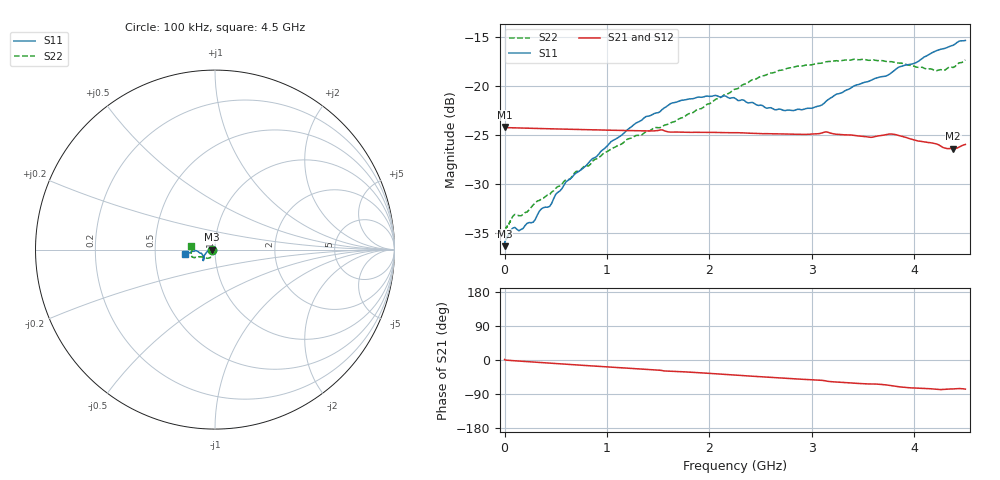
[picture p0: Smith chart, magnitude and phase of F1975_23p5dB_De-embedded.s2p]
! Integrated Device Technology
! Corporate Headquarters
! 6024 Silver Creek Valley Road
! San Jose, CA 95138  USA
! Phone:  1-408-284-8200
! Toll Free:  1-800-223-1366
! Webpage:  http://www.idt.com/
! Timing and RF Division
! 515 Groton Road, Suite 102
! Westford, MA 01886-6024
! Device:  F1975
! Description: 6-bit, 75 ohm, 0.5 dB Digital Step Attenuator
! Frequency:  5.0 MHz -  3.00 GHz
! Package:  4x4 mm QFN Plastic Package: 20 pin
! Ports:  2 RF, 11 DC
!  Pin  1  = D5 (16 dB)
!  Pin  2  = RF1  =  Port 1
!  Pin  3  = Serial Data In (DATA)
!  Pin  4  = Serial Clock (CLK)
!  Pin  5  = Serial Latch Enable (LE)
!  Pin  6  = VDD
!  Pin  7  = NC
!  Pin  8  = NC
!  Pin  9  = NC
!  Pin 10  = GND
!  Pin 11  = GND
!  Pin 12  = NC
!  Pin 13  = VMODE
!  Pin 14  = RF2  =  Port 2
!  Pin 15  = D4 (8 dB)
!  Pin 16  = D3 (4 dB)
!  Pin 17  = D2 (2 dB)
!  Pin 18  = NC
!  Pin 19  = D1 (1 dB)
!  Pin 20  = D0 (0.5 dB)
! State:  47
! Atten State:  23.5 dB
! Voltage:  +3.30 Volts
! Current:  0.563 mA
! Data:  The device was measured on a F1975 evaluation board which has
!  individual transmission lines to the RF pins.  Data was collected
!  using a calibrated network analyzer.  The evaluation board was
!  de-embedded using Automatic Fixture Removal (AFR).
!  The reference plane is the edge of the package pin.
! Misc:
!  Action Tracker AT0415
! Date Measured:  2018-02-08
! Date:  2018-03-26  MJV
! Note:
!  Integrated Device Technology supplies this data as a sample of measured
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# GHz S dB R 75
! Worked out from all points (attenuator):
!   291 points, 100 kHz to 4.5 GHz, reference 75 ohm
!   highest |S21| = -24.14 dB at 100 kHz (marker M1); lowest = -26.4 dB at 4.38 GHz (marker M2)
!   lowest |S11| = -36.3 dB at 100 kHz (marker M3), VSWR 1.03, Z = 72.7 - j0.00568 ohm
!   |S11| at or under -10 dB: start of sweep to end of sweep
!   |S22| runs from -35.3 to -17.2 dB; largest |S21 - S12| = 0.00017
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0.0001  -36.29 -179.9  -24.14 1.2  -24.14 1.2  -35.28 -178.9
0.002  -35.87 -178.5  -24.17 0.9  -24.18 0.9  -34.86 -177.3
0.009  -35.72 -178.6  -24.20 -0.1  -24.19 -0.2  -34.48 -175.7
0.1  -34.38 -175.3  -24.23 -2.1  -24.23 -2.1  -33.06 -161.4
0.16  -34.59 -177.4  -24.25 -3.2  -24.25 -3.2  -33.20 -153.6
0.28  -33.85 179.5  -24.28 -5.5  -24.28 -5.5  -32.08 -144.3
0.36  -32.49 179.6  -24.30 -6.9  -24.30 -6.9  -31.48 -136.3
0.44  -32.24 180.0  -24.32 -8.3  -24.32 -8.3  -31.06 -130.7
0.6  -29.74 -176.3  -24.37 -11.2  -24.37 -11.2  -29.52 -125.7
0.76  -28.40 -169.5  -24.40 -14.0  -24.40 -14.0  -28.32 -123.0
1.28  -23.76 -152.8  -24.53 -23.0  -24.53 -23.0  -25.02 -122.6
1.52  -22.56 -144.7  -24.44 -27.1  -24.44 -27.1  -24.20 -129.2
1.62  -21.76 -142.9  -24.66 -29.4  -24.66 -29.4  -23.73 -132.5
1.88  -21.12 -138.9  -24.69 -33.3  -24.69 -33.3  -22.36 -144.2
2.26  -21.29 -137.8  -24.73 -39.9  -24.73 -39.9  -20.26 -155.3
2.64  -22.39 -147.1  -24.84 -46.4  -24.83 -46.5  -18.57 -158.3
3.02  -22.16 -163.7  -24.85 -52.5  -24.84 -52.5  -17.74 -160.8
3.42  -19.92 -175.1  -25.01 -61.3  -25.01 -61.3  -17.23 -166.3
3.76  -18.75 -175.5  -24.86 -67.0  -24.86 -67.0  -17.49 -172.7
4.2  -16.44 -172.4  -25.83 -76.8  -25.83 -76.7  -18.40 175.4
4.38  -15.82 -170.4  -26.35 -76.4  -26.35 -76.3  -18.08 173.1
4.5  -15.32 -172.0  -25.92 -76.9  -25.92 -76.9  -17.30 170.6
